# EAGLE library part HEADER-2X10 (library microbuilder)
PIN HEADER
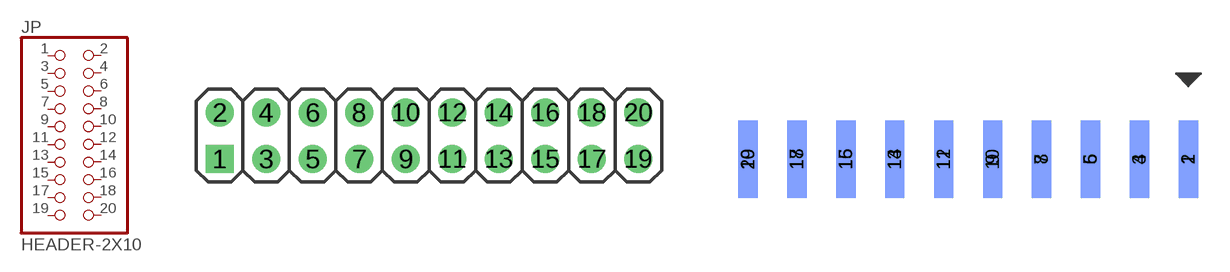
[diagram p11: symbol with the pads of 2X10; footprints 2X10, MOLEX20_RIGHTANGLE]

Designator prefix JP

## HEADER-2X10  [2X10]
1  1  pas
2  2  pas
3  3  pas
4  4  pas
5  5  pas
6  6  pas
7  7  pas
8  8  pas
9  9  pas
10  10  pas
11  11  pas
12  12  pas
13  13  pas
14  14  pas
15  15  pas
16  16  pas
17  17  pas
18  18  pas
19  19  pas
20  20  pas

## HEADER-2X10MOLEX20_SIDE  [MOLEX20_RIGHTANGLE]
Pads as for 2X10

## Footprint 2X10 (pad centres in mm)
PIN HEADER
drill 1 square: 1 -11.43,-1.27
drill 1: 2 -11.43,1.27; 3 -8.89,-1.27; 4 -8.89,1.27; 5 -6.35,-1.27; 6 -6.35,1.27; 7 -3.81,-1.27; 8 -3.81,1.27; 9 -1.27,-1.27; 10 -1.27,1.27; 11 1.27,-1.27; 12 1.27,1.27; 13 3.81,-1.27; 14 3.81,1.27; 15 6.35,-1.27; 16 6.35,1.27; 17 8.89,-1.27; 18 8.89,1.27; 19 11.43,-1.27; 20 11.43,1.27

## Footprint MOLEX20_RIGHTANGLE (pad centres in mm)
Molex 20 Pin Header Footprint designed to mount connector on edge of board, one row on top layer, one row on bottom layer
smd 1 x 4: 1 11.43,0; 3 8.89,0; 5 6.35,0; 7 3.81,0; 9 1.27,0; 11 -1.27,0; 13 -3.81,0; 15 -6.35,0; 17 -8.89,0; 19 -11.43,0
smd 1 x 4 bottom: 2 11.43,0; 4 8.89,0; 6 6.35,0; 8 3.81,0; 10 1.27,0; 12 -1.27,0; 14 -3.81,0; 16 -6.35,0; 18 -8.89,0; 20 -11.43,0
